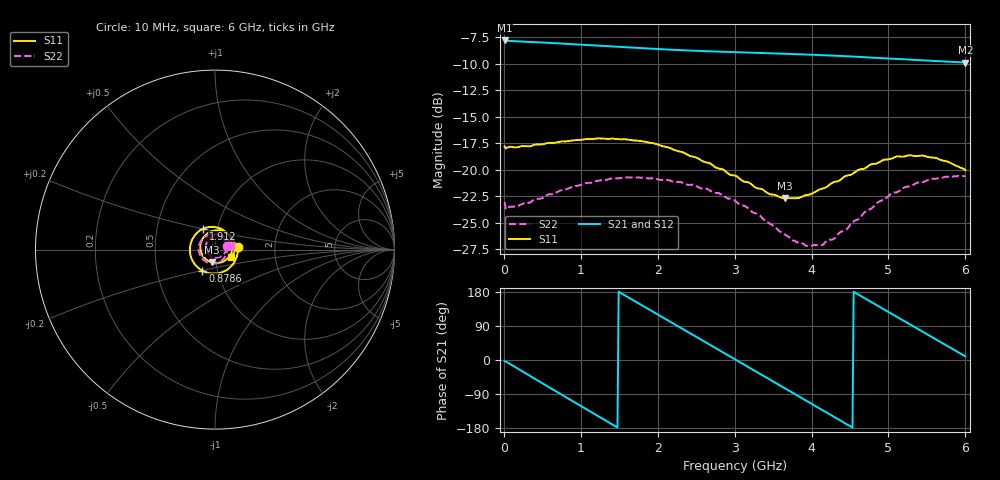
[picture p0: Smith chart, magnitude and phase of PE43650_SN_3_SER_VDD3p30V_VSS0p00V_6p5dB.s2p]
!Keysight Technologies,N5245B,MY57181451,A.13.50.07
!Date: Tuesday, May 07, 2019 07:59:57
!Correction: S11(Full 2 Port(1,2))
!S21(Full 2 Port(1,2))
!S12(Full 2 Port(1,2))
!S22(Full 2 Port(1,2))
!S2P File: Measurements: S11, S21, S12, S22:
# Hz S  dB  R 50
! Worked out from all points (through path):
!   401 points, 10 MHz to 6 GHz, reference 50 ohm
!   highest |S21| = -7.82 dB at 10 MHz (marker M1); lowest = -9.9 dB at 6 GHz (marker M2)
!   group delay of S21, straight-line fit = 328 ps
!   lowest |S11| = -22.7 dB at 3.649 GHz (marker M3), VSWR 1.16, Z = 47.8 - j6.83 ohm
!   |S11| at or under -10 dB: start of sweep to end of sweep
!   |S22| runs from -27.2 to -20.6 dB; largest |S21 - S12| = 0.003
!   S11 on the Smith chart (normalised r, x): 10 MHz: 1.29, +0.04; 878.5 MHz: 0.85, -0.20; 1.912 GHz: 0.86, +0.20; 6 GHz: 1.20, -0.10
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1e7  -17.81 6.5  -7.82 -3.3  -7.87 -3.3  -23.07 16.8
2.34625e8  -17.78 -34.1  -7.92 -29.2  -7.97 -29.2  -23.25 -34.0
4.892e8  -17.63 -69.4  -8.01 -60.0  -8.06 -60.0  -22.71 -69.4
8.7855e8  -17.26 -120.6  -8.15 -106.8  -8.21 -106.9  -21.65 -118.6
1.013325e9  -17.18 -137.4  -8.22 -123.0  -8.26 -123.0  -21.38 -134.2
1.462575e9  -17.11 169.6  -8.40 -176.4  -8.46 -176.4  -20.82 178.5
1.911825e9  -17.48 119.2  -8.59 130.5  -8.65 130.5  -20.82 134.9
2.01665e9  -17.66 107.8  -8.63 118.1  -8.69 118.1  -20.93 125.2
2.241275e9  -18.21 82.9  -8.71 91.7  -8.77 91.7  -21.19 103.9
2.4659e9  -18.79 57.2  -8.78 65.3  -8.84 65.3  -21.45 82.7
2.750425e9  -19.79 24.5  -8.86 31.9  -8.91 32.0  -22.19 54.6
3.005e9  -20.57 -8.1  -8.92 2.0  -8.97 2.0  -22.93 28.0
3.3045e9  -21.78 -50.0  -8.99 -33.3  -9.04 -33.2  -24.26 -7.8
3.648925e9  -22.72 -103.8  -9.07 -73.9  -9.12 -73.9  -26.11 -55.7
4.008325e9  -22.26 -162.1  -9.17 -116.3  -9.22 -116.3  -27.16 -117.0
4.277875e9  -21.22 158.4  -9.25 -148.2  -9.30 -148.1  -26.55 -163.8
4.517475e9  -20.46 126.0  -9.33 -176.5  -9.38 -176.4  -25.06 158.3
4.757075e9  -19.56 96.6  -9.43 155.2  -9.48 155.4  -23.75 128.3
5.01165e9  -19.02 68.5  -9.52 125.3  -9.57 125.5  -22.42 98.5
5.4609e9  -18.70 23.0  -9.69 72.6  -9.74 72.8  -21.14 55.4
5.745425e9  -19.21 -3.0  -9.81 39.3  -9.85 39.4  -20.67 31.1
6e9  -20.04 -24.2  -9.90 9.6  -9.94 9.6  -20.62 11.6
